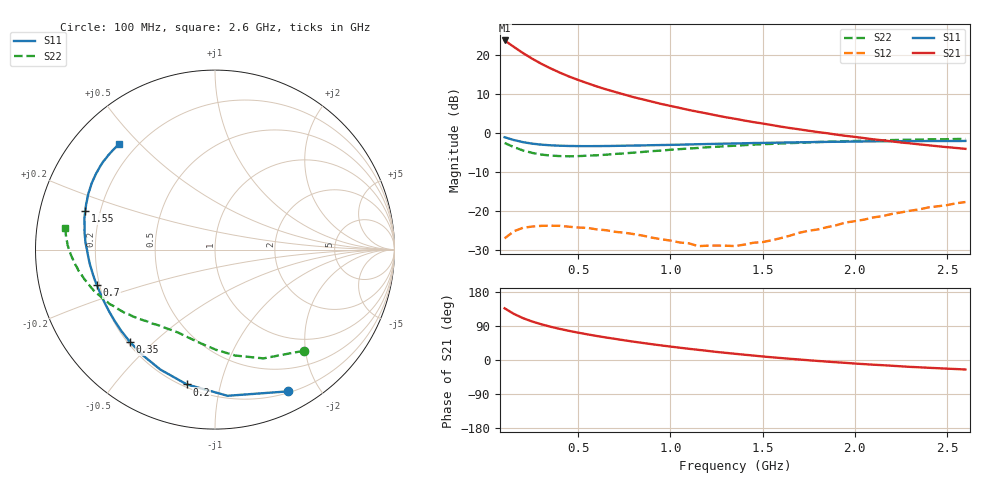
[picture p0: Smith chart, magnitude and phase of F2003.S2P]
!  POLYFET RF DEVICES
!  S PARAMETERS FOR
!  F2003 (Each Side)
!  VDS=28, IDQ=200mA
! Date: Mon Aug  5 14:30:38 1991
# MHZ S MA R 50
!  FREQ  S11  S11 ANG  S21  S21 ANG  S12  S12 ANG  S22  S22 ANG
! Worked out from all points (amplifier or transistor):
!   51 points, 100 MHz to 2.6 GHz, reference 50 ohm
!   highest |S21| = 23.8 dB at 100 MHz (marker M1)
!   |S21| within 3 dB of that: start of sweep to 192.6 MHz
!   unconditionally stable (mu >= 1): 866 MHz to 1.912 GHz
!   at 500 MHz: K = 0.48, MSG = 18.9 dB, |S12| = -24.2 dB
!   at 1.35 GHz: K = 1.76, MAG = 11.2 dB, |S12| = -28.9 dB
!   at 2.6 GHz: K = 0.55, MSG = 6.8 dB, |S12| = -17.6 dB
!   S11 on the Smith chart (normalised r, x): 100 MHz: 0.22, -1.61; 200 MHz: 0.22, -0.79; 350 MHz: 0.21, -0.42; 700 MHz: 0.19, -0.14; 1.55 GHz: 0.14, +0.14; 2.6 GHz: 0.14, +0.43
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100  0.8875 -62.9  15.41 136.4  0.04493 50.8  0.7491 -48.8
150  0.8175 -85.1  12.76 121.7  0.05533 37.7  0.6634 -66.0
200  0.7674 -101.8  10.62 110.4  0.06145 28.7  0.6012 -79.1
250  0.7345 -114.5  8.99 101.5  0.06374 21.1  0.5592 -89.2
300  0.7129 -124.5  7.73 94.2  0.06503 16.2  0.5319 -97.2
350  0.6995 -132.5  6.756 87.7  0.06535 12.2  0.5169 -103.7
400  0.6913 -139.1  5.96 82.0  0.06502 8.4  0.5089 -109.3
450  0.6858 -144.6  5.317 76.9  0.06337 5.9  0.5059 -114.0
500  0.6832 -149.3  4.801 72.1  0.06186 4.1  0.5088 -118.1
550  0.6825 -153.4  4.36 67.7  0.06127 0.3  0.5151 -121.5
600  0.6834 -157.1  3.969 63.4  0.05853 -0.4  0.5213 -124.9
650  0.6848 -160.4  3.646 59.4  0.05719 -0.8  0.53 -127.9
700  0.6877 -163.4  3.372 55.7  0.05452 -2.2  0.5426 -130.8
800  0.6942 -168.7  2.894 48.3  0.05099 -4.1  0.5634 -135.9
950  0.7052 -175.5  2.369 38.5  0.04378 -1.0  0.5991 -142.8
1100  0.7174 178.6  1.982 29.5  0.03885 7.0  0.6365 -149.0
1250  0.731 173.2  1.686 21.3  0.03636 17.7  0.67 -154.8
1350  0.7381 169.8  1.53 16.4  0.03581 27.4  0.6915 -158.2
1550  0.7541 163.5  1.271 7.2  0.04255 43.1  0.73 -164.6
1800  0.7717 156.1  1.033 -2.5  0.05851 53.6  0.7701 -171.3
2200  0.7895 144.5  0.7866 -15.1  0.09226 53.2  0.8161 179.4
2600  0.7958 132.4  0.63 -25.1  0.1314 48.1  0.8431 171.8
